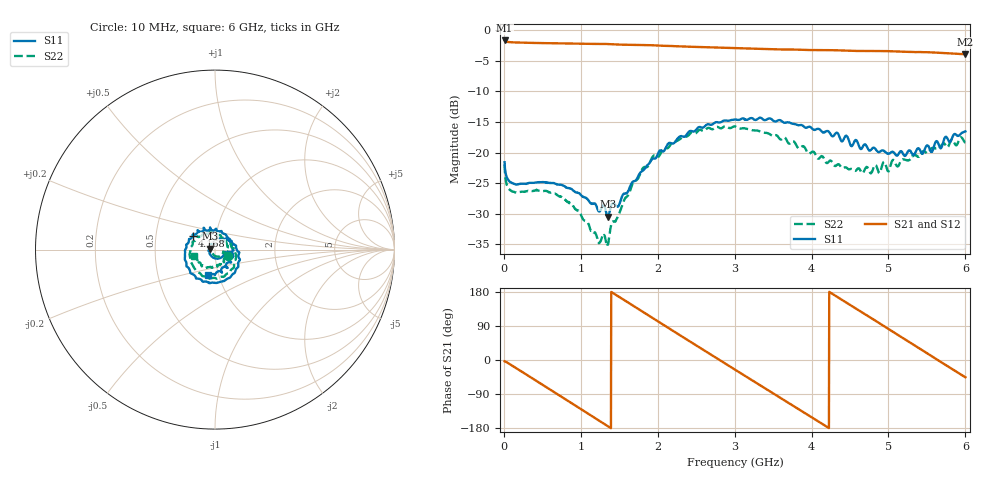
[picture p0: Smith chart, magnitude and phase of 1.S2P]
!Agilent Technologies,E5071C,MY46316741,A.11.02
!Date: Thu Jul 30 16:11:05 2020
!Data & Calibration Information:
!Freq	S11:SOLT4(ON)	S21:SOLT4(ON)	S12:SOLT4(ON)	S22:SOLT4(ON)
!PortZ  Port1:50+j0  Port2:50+j0
!Above PortZ is port z conversion or system Z0 setting when saving the data.
!When reading, reference impedance value at option line is always used.
# Hz S dB R 50
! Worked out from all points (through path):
!   1561 points, 10 MHz to 6 GHz, reference 50 ohm
!   highest |S21| = -1.71 dB at 10 MHz (marker M1); lowest = -4.0 dB at 6 GHz (marker M2)
!   group delay of S21, straight-line fit = 354 ps
!   lowest |S11| = -30.5 dB at 1.35 GHz (marker M3), VSWR 1.06, Z = 47.1 + j0.462 ohm
!   |S11| at or under -10 dB: start of sweep to end of sweep
!   |S22| runs from -35.3 to -15.7 dB; largest |S21 - S12| = 0.01
!   S11 on the Smith chart (normalised r, x): 10 MHz: 1.17, -0.07; 4.168 GHz: 0.77, +0.12; 6 GHz: 0.88, -0.26
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1e7  -21.59 -20.0  -1.71 -3.4  -1.71 -3.4  -21.98 -24.6
1.136731e8  -24.99 -13.5  -2.02 -15.5  -2.02 -15.5  -26.35 -13.8
5.514038e8  -24.91 -44.4  -2.15 -71.6  -2.15 -71.7  -26.27 -42.5
7.779487e8  -25.42 -71.0  -2.20 -100.7  -2.19 -100.8  -27.44 -67.8
1.012173e9  -27.07 -107.7  -2.24 -130.8  -2.24 -131.0  -30.45 -105.2
1.350071e9  -30.49 170.6  -2.30 -174.4  -2.29 -174.6  -34.94 138.4
1.65341e9  -25.21 89.5  -2.44 146.8  -2.43 146.6  -25.77 65.6
2.006667e9  -20.09 30.7  -2.56 101.3  -2.55 101.2  -20.69 12.0
2.263929e9  -17.64 -5.7  -2.67 68.6  -2.66 68.1  -18.03 -22.1
2.563429e9  -15.89 -39.1  -2.79 30.6  -2.79 30.2  -16.32 -59.9
2.786135e9  -15.08 -64.2  -2.88 2.3  -2.87 1.9  -15.86 -87.7
3.005e9  -14.61 -87.6  -2.95 -25.5  -2.95 -26.0  -15.74 -115.8
3.269942e9  -14.70 -116.0  -3.08 -58.9  -3.07 -59.3  -16.40 -148.8
3.504167e9  -14.81 -140.6  -3.15 -88.5  -3.13 -89.0  -17.24 179.3
3.742231e9  -15.27 -165.6  -3.20 -118.4  -3.19 -119.0  -18.25 145.0
4.007173e9  -16.09 168.1  -3.28 -151.9  -3.26 -152.6  -19.88 107.7
4.168442e9  -16.63 147.9  -3.31 -172.3  -3.29 -172.9  -21.13 83.7
4.636891e9  -19.40 96.3  -3.44 128.3  -3.43 127.6  -22.95 8.0
5.001667e9  -20.20 41.5  -3.46 81.7  -3.46 80.9  -23.09 -43.9
5.516192e9  -18.92 -37.7  -3.64 15.9  -3.63 15.1  -20.04 -105.2
5.742737e9  -17.43 -73.3  -3.79 -13.2  -3.78 -14.0  -18.83 -132.0
6e9  -16.56 -106.2  -3.96 -45.6  -3.94 -46.5  -18.36 -163.7
